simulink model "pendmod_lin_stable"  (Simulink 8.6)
settings: Solver=ode1  StartTime=0.0  StopTime=100  FixedStep=0.001  RelTol=1e-3
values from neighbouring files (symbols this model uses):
  g = 9.81    [test_omega.m]
  l = 0.39    [test_omega.m]
  m = 0.23    [test_omega.m]
undefined symbols (not defined in the file or in its folder): d, d0, d1, d2, d3, In

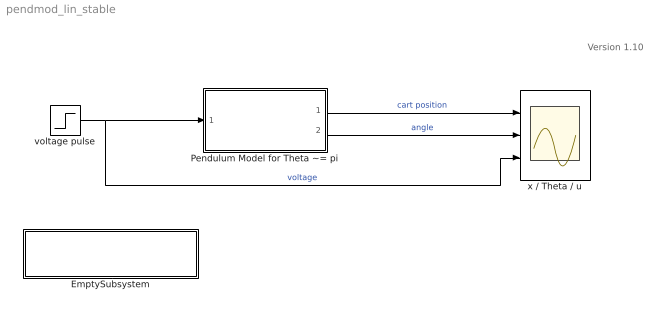
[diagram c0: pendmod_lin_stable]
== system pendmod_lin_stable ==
  note: Version 1.10
  EmptySubsystem : Subsystem
  Pendulum Model for Theta ~= pi : Subsystem
  voltage pulse : Step  Time=0.01  Before=0.1  After=0  SampleTime=0
  x / Theta / u : Scope  NumInputPorts=3
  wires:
  voltage pulse/1 -> Pendulum Model for Theta ~= pi/1(u), x / Theta / u/3  "voltage"
  Pendulum Model for Theta ~= pi/1(x) -> x / Theta / u/1  "cart position"
  Pendulum Model for Theta ~= pi/2(Theta) -> x / Theta / u/2  "angle"

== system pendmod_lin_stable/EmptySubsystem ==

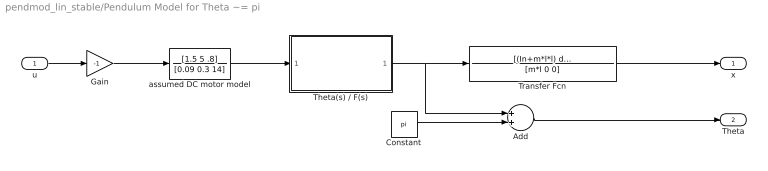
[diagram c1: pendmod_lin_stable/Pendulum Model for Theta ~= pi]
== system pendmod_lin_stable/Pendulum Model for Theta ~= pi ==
  u : Inport
  Add : Sum
  Constant : Constant  Value=pi
  Gain : Gain  Gain=-1
  Theta(s) / F(s) : Subsystem
  Transfer Fcn : TransferFcn  Tag=s  Numerator=[(In+m*l*l) d -m*g*l]  Denominator=[m*l 0 0]
  assumed DC motor model : TransferFcn  Numerator=[1.5 5 .8]  Denominator=[0.09 0.3 14]
  x : Outport
  Theta : Outport  Port=2
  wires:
  Theta(s) / F(s)/1(Out1) -> Transfer Fcn/1, Add/1
  Transfer Fcn/1 -> x/1
  assumed DC motor model/1 -> Theta(s) / F(s)/1(F)
  u/1 -> Gain/1
  Gain/1 -> assumed DC motor model/1
  Add/1 -> Theta/1
  Constant/1 -> Add/2

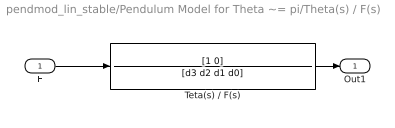
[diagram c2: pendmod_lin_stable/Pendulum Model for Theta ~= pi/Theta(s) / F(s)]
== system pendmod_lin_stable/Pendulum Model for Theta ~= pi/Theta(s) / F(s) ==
  F : Inport
  Teta(s) / F(s) : TransferFcn  Numerator=[1 0]  Denominator=[d3 d2 d1 d0]
  Out1 : Outport
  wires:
  F/1 -> Teta(s) / F(s)/1
  Teta(s) / F(s)/1 -> Out1/1
